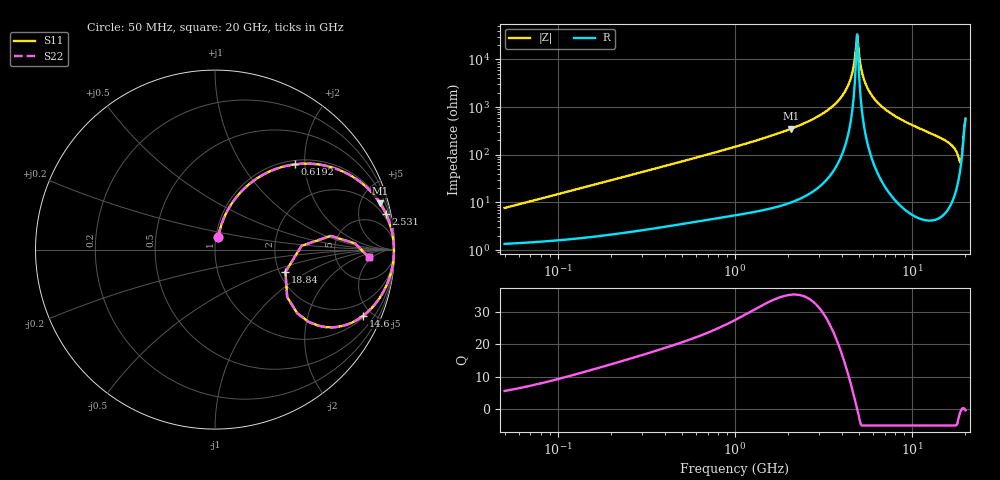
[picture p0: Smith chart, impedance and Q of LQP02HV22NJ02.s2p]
!Murata Part Number: LQP02HV22NJ02
!These Parameters are Measured in Series Mode Connection
!  o--[Z]--o
!Port1  Port2
!  o-------o
!Freq. Start=50[MHz] Stop=20[GHz], 401[Steps]
# Hz S RI R 50
!Freq.(Hz) S11(Real) S11(Imag) S21(Real) S21(Imag) S12(Real) S12(Imag) S22(Real) S22(Imag)
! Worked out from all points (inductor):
!   401 points, 50 MHz to 20 GHz, reference 50 ohm
!   read as one part in series: L = 23.8 nH near 51.52 MHz
!   highest Q = 35.2 at 2.083 GHz (marker M1), where L = 27 nH
!   self-resonance near 4.893 GHz
!   S11 on the Smith chart (normalised r, x): 50 MHz: 1.03, +0.15; 619.2 MHz: 1.08, +1.78; 2.531 GHz: 1.28, +9.58; 14.6 GHz: 1.10, -4.44; 18.84 GHz: 2.16, -0.65; 20 GHz: 12, -4
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5e7  0.0187 0.0729  0.9813 -0.0729  0.9813 -0.0729  0.0187 0.0729
1.364002e8  0.0543 0.1864  0.9457 -0.1864  0.9457 -0.1864  0.0543 0.1864
3.721004e8  0.2364 0.3983  0.7636 -0.3983  0.7636 -0.3983  0.2364 0.3983
6.192061e8  0.446 0.4752  0.554 -0.4752  0.554 -0.4752  0.446 0.4752
1e9  0.6762 0.45  0.3238 -0.45  0.3238 -0.45  0.6762 0.45
2.083303e9  0.9196 0.258  0.0804 -0.258  0.0804 -0.258  0.9196 0.258
2.531158e9  0.953 0.1977  0.047 -0.1977  0.047 -0.1977  0.953 0.1977
2.728004e9  0.9629 0.1746  0.0371 -0.1746  0.0371 -0.1746  0.9629 0.1746
3.466789e9  0.9854 0.1021  0.0146 -0.1021  0.0146 -0.1021  0.9854 0.1021
4.087748e9  0.9937 0.0533  0.00629 -0.0533  0.00629 -0.0533  0.9937 0.0533
4.472136e9  0.9961 0.0268  0.0039 -0.0268  0.0039 -0.0268  0.9961 0.0268
4.81993e9  0.997 0.00474  0.00302 -0.00474  0.00302 -0.00474  0.997 0.00474
4.89267e9  0.997 0.000328  0.00297 -0.000328  0.00297 -0.000328  0.997 0.000328
5.041459e9  0.997 -0.00851  0.00299 0.00851  0.00299 0.00851  0.997 -0.00851
5.273168e9  0.9967 -0.0218  0.00331 0.0218  0.00331 0.0218  0.9967 -0.0218
5.598765e9  0.9957 -0.0396  0.00432 0.0396  0.00432 0.0396  0.9957 -0.0396
6.311513e9  0.9916 -0.0756  0.00839 0.0756  0.00839 0.0756  0.9916 -0.0756
7.442007e9  0.9811 -0.1265  0.0189 0.1265  0.0189 0.1265  0.9811 -0.1265
1.460232e10  0.8262 -0.3679  0.1738 0.3679  0.1738 0.3679  0.8262 -0.3679
1.747767e10  0.6173 -0.4318  0.3827 0.4318  0.3827 0.4318  0.6173 -0.4318
1.88369e10  0.3924 -0.1242  0.6076 0.1242  0.6076 0.1242  0.3924 -0.1242
2e10  0.8567 -0.0434  0.1433 0.0434  0.1433 0.0434  0.8567 -0.0434
